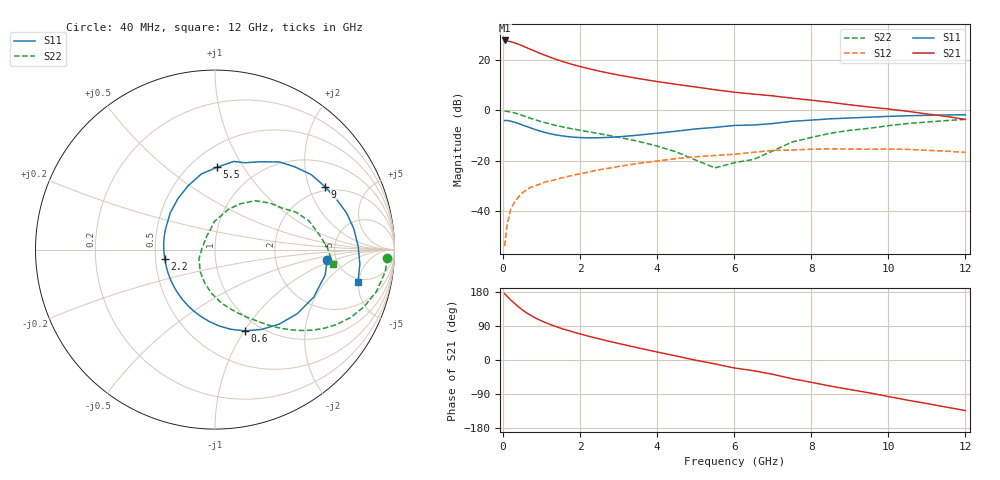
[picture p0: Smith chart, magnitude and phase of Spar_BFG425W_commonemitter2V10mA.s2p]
! Filename: 210bfg425.001
! BFG425W Field C1
! V1=8.464E-001V,V2=2.000E+000V, I1=1.354E-004A, I2=9.990E-003A
# GHz  S  MA  R 50
!  S11  S21  S12  S22
!Freq(GHz)  Mag  Ang  Mag  Ang  Mag  Ang  Mag  Ang
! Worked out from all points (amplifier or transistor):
!   44 points, 40 MHz to 12 GHz, reference 50 ohm
!   highest |S21| = 27.8 dB at 40 MHz (marker M1)
!   |S21| within 3 dB of that: start of sweep to 633.8 MHz
!   unconditionally stable (mu >= 1): 1.849 GHz to end of sweep
!   at 700 MHz: K = 0.53, MSG = 27.6 dB, |S12| = -30.8 dB
!   at 2.4 GHz: K = 1.10, MAG = 18.0 dB, |S12| = -23.9 dB
!   at 12 GHz: K = 1.39, MAG = 2.8 dB, |S12| = -16.7 dB
!   lowest NFmin = 1.40 dB at 900 GHz
!   S11 on the Smith chart (normalised r, x): 40 MHz: 4.21, -0.81; 600 MHz: 0.85, -1.01; 2.2 GHz: 0.56, -0.06; 5.5 GHz: 0.66, +0.77; 9 GHz: 1.84, +2.57; 12 GHz: 4.46, -4.88
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0.04  0.628 -5.3  24.55 174.9  0.002 76.5  0.961 -2.7
0.2  0.61 -25.8  23.14 158.4  0.011 76.9  0.929 -14.6
0.3  0.581 -37.9  21.98 149.2  0.015 71.9  0.889 -21.1
0.4  0.548 -49.3  20.65 140.4  0.019 66.7  0.843 -26.8
0.5  0.514 -60.0  19.26 132.2  0.023 62.7  0.794 -31.8
0.6  0.482 -69.8  17.83 125.2  0.026 59.6  0.747 -36.0
0.8  0.425 -87.2  15.32 113.2  0.031 54.7  0.663 -42.8
0.9  0.401 -94.9  14.23 108.0  0.033 53.0  0.627 -45.6
1  0.38 -102.2  13.23 103.2  0.035 51.5  0.595 -48.1
1.2  0.347 -115.8  11.55 94.7  0.039 49.2  0.542 -52.5
1.4  0.323 -128.0  10.2 87.3  0.043 47.4  0.496 -56.3
1.6  0.306 -139.5  9.1 80.6  0.047 45.9  0.46 -59.7
2.2  0.285 -169.3  6.812 63.4  0.059 41.2  0.378 -69.8
3  0.298 158.0  5.037 43.6  0.077 33.5  0.293 -84.2
3.5  0.322 140.9  4.307 32.2  0.088 27.7  0.244 -94.6
4.5  0.386 112.7  3.293 10.4  0.11 14.2  0.149 -123.4
5.5  0.459 88.6  2.574 -10.4  0.127 -0.7  0.072 171.6
6.5  0.512 70.9  2.109 -28.3  0.147 -12.1  0.106 106.7
8.5  0.68 37.9  1.445 -68.9  0.172 -48.5  0.352 50.7
9  0.706 29.8  1.291 -77.9  0.17 -56.7  0.402 40.1
10.5  0.782 8.6  0.959 -106.0  0.168 -83.3  0.548 16.9
12  0.817 -12.9  0.661 -133.4  0.146 -113.0  0.663 -7.1
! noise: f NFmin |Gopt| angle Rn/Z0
900  1.4  0.02  -63.9  0.19
2000  1.6  0.06  137.4  0.19
